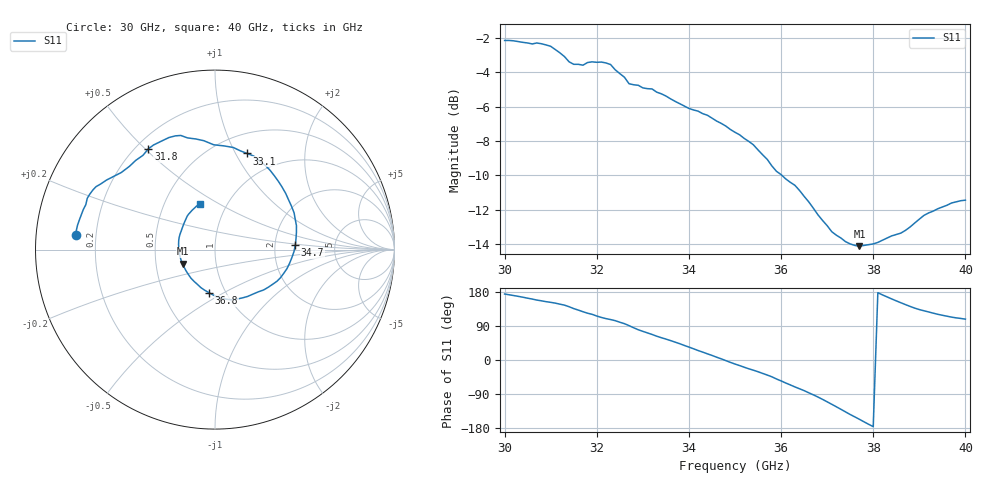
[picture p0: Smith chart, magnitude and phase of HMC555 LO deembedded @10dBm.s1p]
!Hittite Microwave Corporation
!20 Alpha Road
!Chelmsford, MA 01824
!Tel: 978-250-3343
!Fax: 978-250-3373
!Device: HMC555, 32-38GHz, I/Q Mixer
!Misc: LO Return Loss with 10 dBm, Data includes one K connector, Room
# MHZ S MA R 50
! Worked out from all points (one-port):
!   101 points, 30 GHz to 40 GHz, reference 50 ohm
!   lowest |S11| = -14.1 dB at 37.7 GHz (marker M1), VSWR 1.49, Z = 34.3 - j5.61 ohm
!   |S11| at or under -10 dB: 36.02 GHz to end of sweep
!   S11 on the Smith chart (normalised r, x): 30 GHz: 0.12, +0.05; 31.8 GHz: 0.25, +0.51; 33.1 GHz: 0.71, +1.12; 34.7 GHz: 2.61, +0.16; 36.8 GHz: 0.84, -0.43; 40 GHz: 0.75, +0.41
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30000  0.78 174.1
30800  0.763 156.1
31000  0.75 152.1
31300  0.7 144.7
31500  0.665 135.7
31800  0.673 123.5
32200  0.671 109.2
32500  0.625 99.7
32700  0.584 90.7
32900  0.578 79.8
33100  0.565 71.5
33400  0.546 58.9
33800  0.511 43.0
34200  0.486 25.0
34700  0.448 3.1
35000  0.422 -10.7
35300  0.397 -23.2
35600  0.363 -35.4
36000  0.318 -55.2
36300  0.296 -71.0
36800  0.243 -97.7
37100  0.217 -116.9
37500  0.2 -143.8
37700  0.197 -156.5
38200  0.205 171.8
38800  0.224 141.4
39400  0.253 120.6
40000  0.268 107.8
